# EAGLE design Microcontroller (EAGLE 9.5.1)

## Sheet 1 of 3: Board to Board Headers
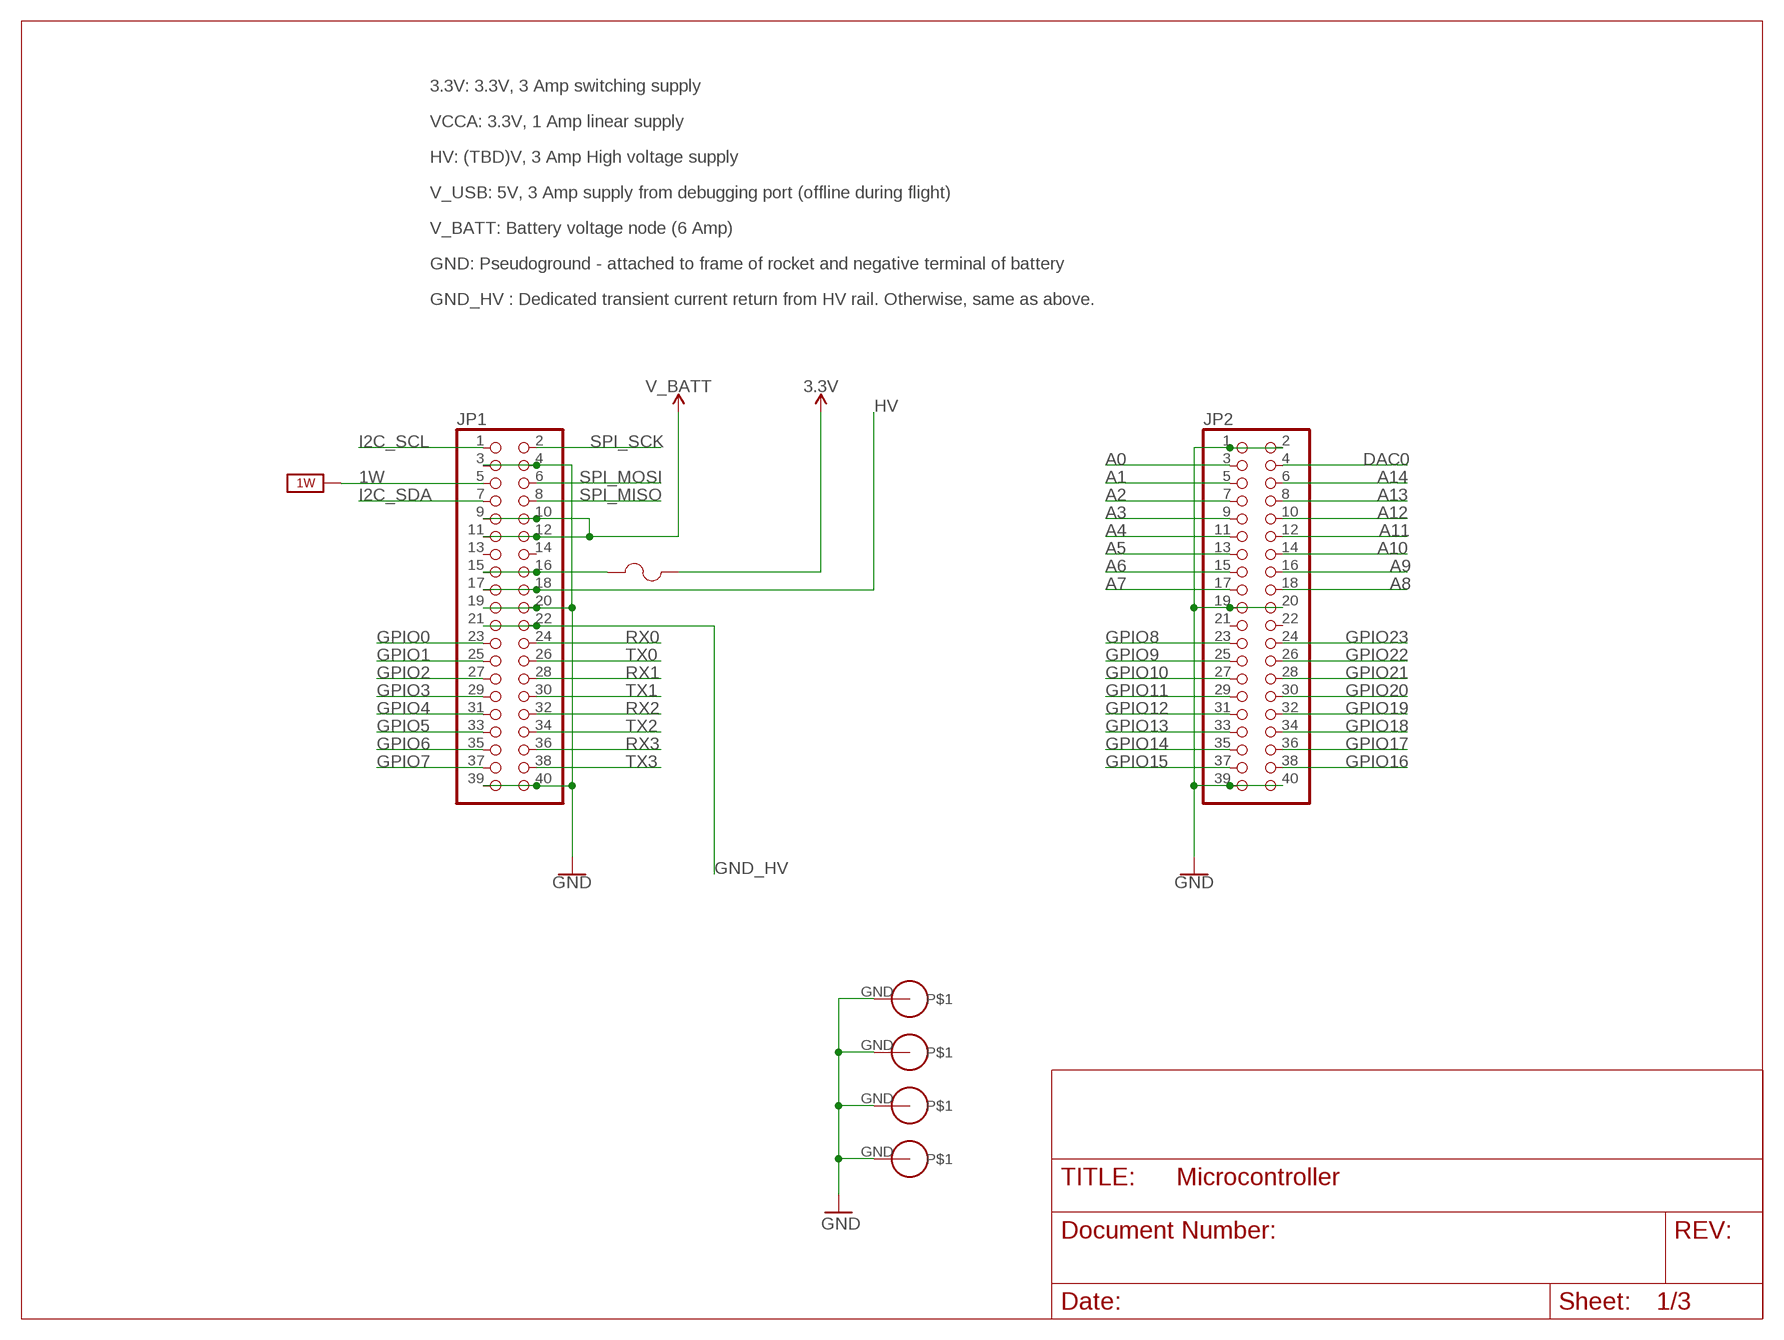
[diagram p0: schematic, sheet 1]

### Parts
F3  0603SFF150F/32-2  [FUS0603_TYCO]
JP1  PINHD-2X20  [2X20]
JP2  PINHD-2X20  [2X20]
U$1  PS/104-MOUNTING-HOLE  [PC/104-MOUNTING-HOLE]
U$2  PS/104-MOUNTING-HOLE  [PC/104-MOUNTING-HOLE]
U$3  PS/104-MOUNTING-HOLE  [PC/104-MOUNTING-HOLE]
U$4  PS/104-MOUNTING-HOLE  [PC/104-MOUNTING-HOLE]

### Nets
1W: JP1.5 ; supply symbol labelled 1W_SUP ; also sheet 3
3.3V: F3.2 ; also sheet 2,3
A0: JP2.3 ; also sheet 2
A1: JP2.5 ; also sheet 2
A2: JP2.7 ; also sheet 2
A3: JP2.9 ; also sheet 2
A4: JP2.11 ; also sheet 2
A5: JP2.13 ; also sheet 2
A6: JP2.15 ; also sheet 2
A7: JP2.17 ; also sheet 2
A8: JP2.18 ; also sheet 2
A9: JP2.16 ; also sheet 2
A10: JP2.14 ; also sheet 2
A11: JP2.12 ; also sheet 2
A12: JP2.10 ; also sheet 2
A13: JP2.8 ; also sheet 2
A14: JP2.6 ; also sheet 2
DAC0: JP2.4 ; also sheet 2
GND: JP1.3 JP1.4 JP1.19 JP1.20 JP1.39 JP1.40 JP2.1 JP2.2 JP2.19 JP2.20 JP2.39 JP2.40 U$1.GND U$2.GND U$3.GND U$4.GND ; also sheet 2,3
GND_HV: JP1.21 JP1.22
GPIO0: JP1.23 ; also sheet 2
GPIO1: JP1.25 ; also sheet 2
GPIO2: JP1.27 ; also sheet 2
GPIO3: JP1.29 ; also sheet 2
GPIO4: JP1.31 ; also sheet 2
GPIO5: JP1.33 ; also sheet 2
GPIO6: JP1.35 ; also sheet 2
GPIO7: JP1.37 ; also sheet 2
GPIO8: JP2.23 ; also sheet 2
GPIO9: JP2.25 ; also sheet 2
GPIO10: JP2.27 ; also sheet 2
GPIO11: JP2.29 ; also sheet 2
GPIO12: JP2.31 ; also sheet 2
GPIO13: JP2.33 ; also sheet 3
GPIO14: JP2.35 ; also sheet 3
GPIO15: JP2.37 ; also sheet 3
GPIO16: JP2.38 ; also sheet 3
GPIO17: JP2.36 ; also sheet 3
GPIO18: JP2.34 ; also sheet 3
GPIO19: JP2.32 ; also sheet 3
GPIO20: JP2.30 ; also sheet 3
GPIO21: JP2.28 ; also sheet 3
GPIO22: JP2.26 ; also sheet 3
GPIO23: JP2.24 ; also sheet 3
HV: JP1.17 JP1.18
I2C_SCL: JP1.1 ; also sheet 2,3
I2C_SDA: JP1.7 ; also sheet 2,3
N$3: F3.1 JP1.15 JP1.16
RX0: JP1.24 ; also sheet 2
RX1: JP1.28 ; also sheet 2
RX2: JP1.32 ; also sheet 2
RX3: JP1.36 ; also sheet 2,3
SPI_MISO: JP1.8 ; also sheet 2,3
SPI_MOSI: JP1.6 ; also sheet 2,3
SPI_SCK: JP1.2 ; also sheet 2,3
TX0: JP1.26 ; also sheet 2
TX1: JP1.30 ; also sheet 2
TX2: JP1.34 ; also sheet 2
TX3: JP1.38 ; also sheet 2,3
V_BATT: JP1.9 JP1.10 JP1.11 JP1.12
Unconnected: JP1.13 JP1.14 JP2.21 JP2.22

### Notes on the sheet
- 3.3V: 3.3V, 3 Amp switching supply
- VCCA: 3.3V, 1 Amp linear supply
- HV: (TBD)V, 3 Amp High voltage supply
- V_USB: 5V, 3 Amp supply from debugging port (offline during flight)
- V_BATT: Battery voltage node (6 Amp)
- GND: Pseudoground - attached to frame of rocket and negative terminal of battery
- GND_HV : Dedicated transient current return from HV rail. Otherwise, same as above.

## Sheet 2 of 3: MCU
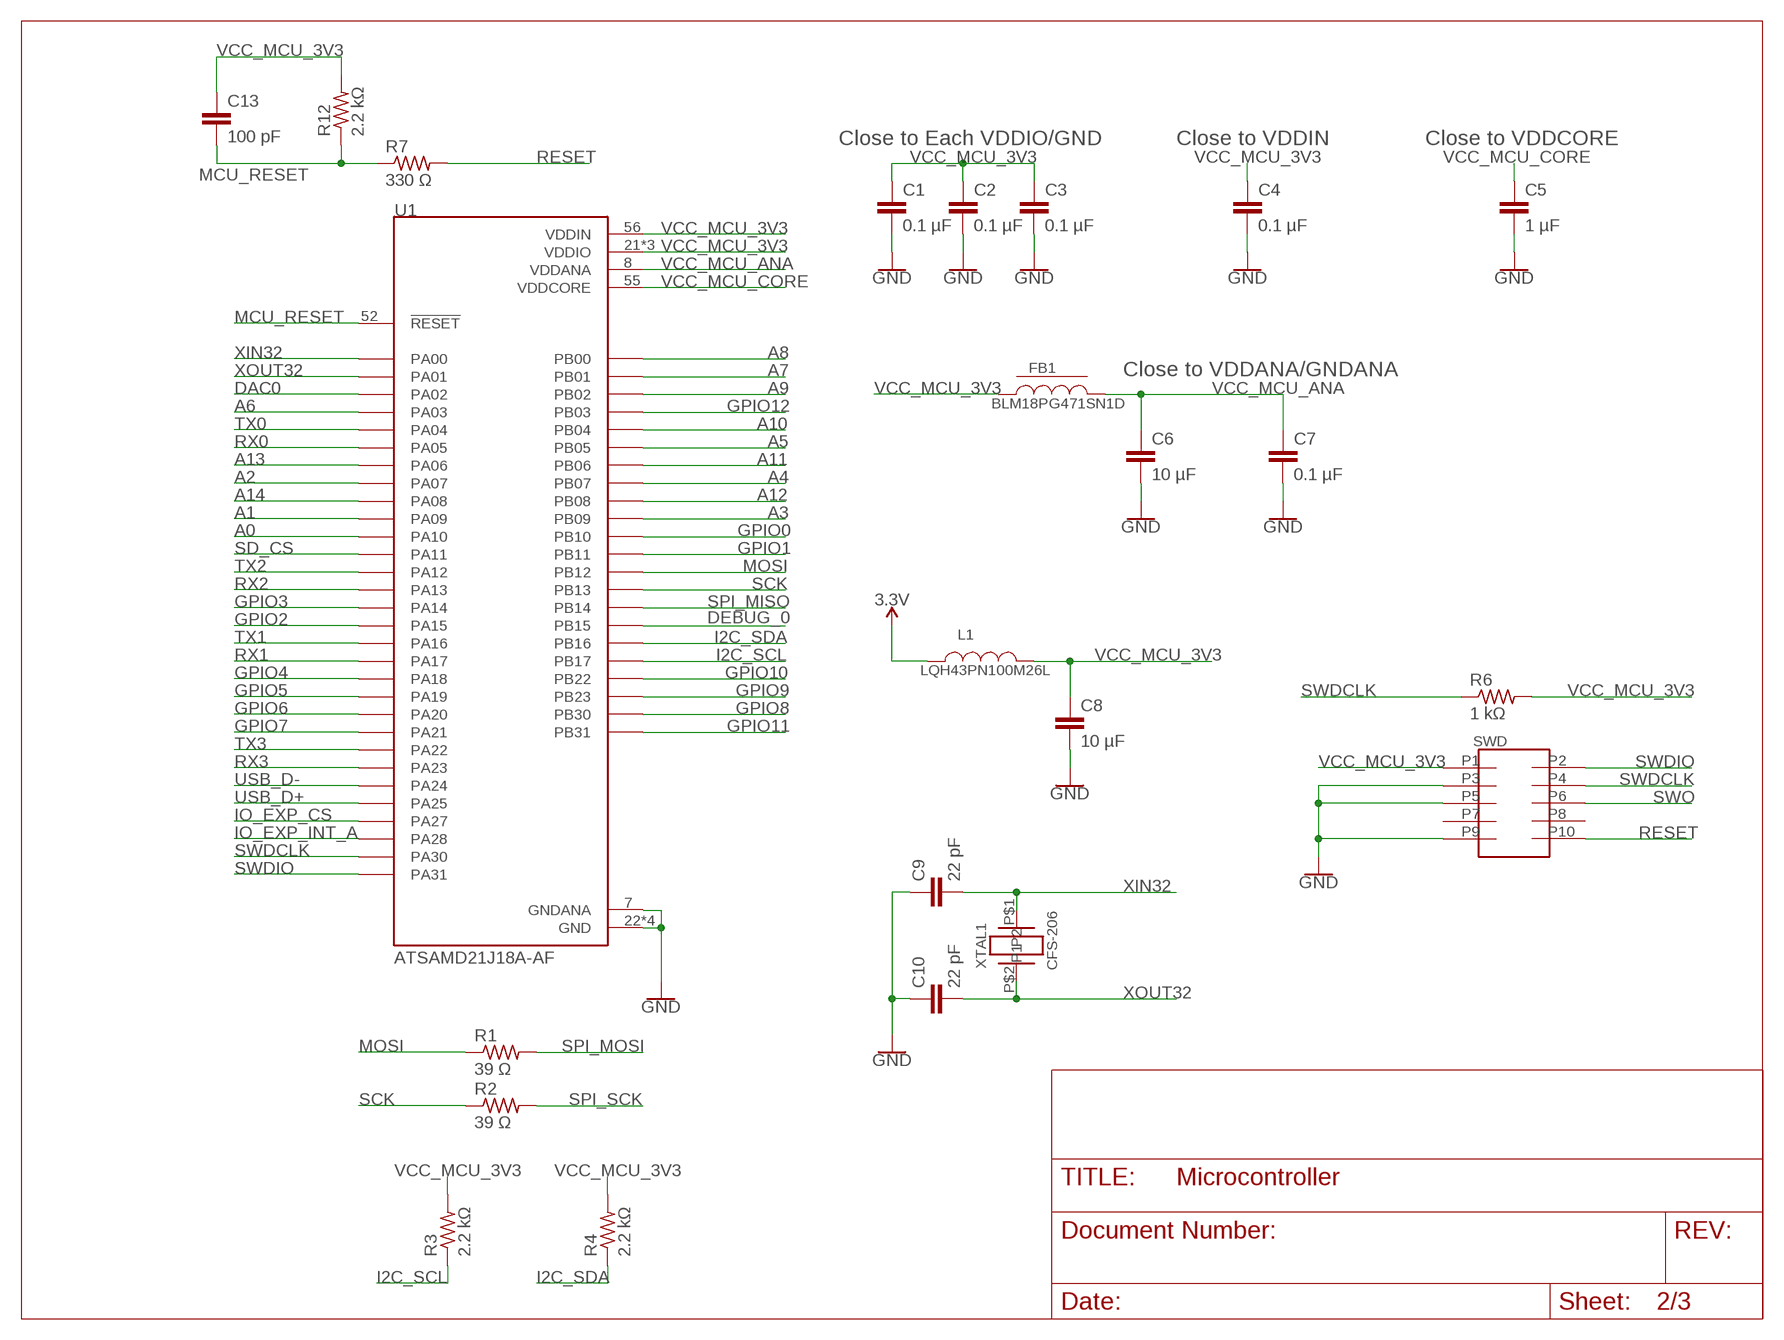
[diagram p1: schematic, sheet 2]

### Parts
C1  0.1 µF  C-EUC0805  [C0805]
C2  0.1 µF  C-EUC0805  [C0805]
C3  0.1 µF  C-EUC0805  [C0805]
C4  0.1 µF  C-EUC0805  [C0805]
C5  1 µF  C-EUC0805  [C0805]
C6  10 µF  C-EUC1206  [C1206]
C7  0.1 µF  C-EUC0805  [C0805]
C8  10 µF  C-EUC1206  [C1206]
C9  22 pF  C-EUC0805  [C0805]
C10  22 pF  C-EUC0805  [C0805]
C13  100 pF  C-EUC0805  [C0805]
FB1  BLM18PG471SN1D  [0603]
L1  LQH43PN100M26L  [LQH43PN100M26L]
R1  39 Ω  R-US_R1206  [R1206]
R2  39 Ω  R-US_R1206  [R1206]
R3  2.2 kΩ  R-US_R1206  [R1206]
R4  2.2 kΩ  R-US_R1206  [R1206]
R6  1 kΩ  R-US_R1206  [R1206]
R7  330 Ω  R-US_R1206  [R1206]
R12  2.2 kΩ  R-US_R1206  [R1206]
SWD  GRPB052VWVN-RC  [GRPB052VWVN-RC]
U1  ATSAMD21J18A-AF  [QFP50P1200X1200X120_64N]
XTAL1  CFS-206  [CFS-206]

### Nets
3.3V: L1.1 ; also sheet 1,3
A0: U1.19(PA10) ; also sheet 1
A1: U1.18(PA09) ; also sheet 1
A2: U1.16(PA07) ; also sheet 1
A3: U1.12(PB09) ; also sheet 1
A4: U1.10(PB07) ; also sheet 1
A5: U1.6(PB05) ; also sheet 1
A6: U1.4(PA03) ; also sheet 1
A7: U1.62(PB01) ; also sheet 1
A8: U1.61(PB00) ; also sheet 1
A9: U1.63(PB02) ; also sheet 1
A10: U1.5(PB04) ; also sheet 1
A11: U1.9(PB06) ; also sheet 1
A12: U1.11(PB08) ; also sheet 1
A13: U1.15(PA06) ; also sheet 1
A14: U1.17(PA08) ; also sheet 1
DAC0: U1.3(PA02) ; also sheet 1
DEBUG_0: U1.28(PB15) ; also sheet 3
GND: C1.2 C2.2 C3.2 C4.2 C5.2 C6.2 C7.2 C8.2 C9.1 C10.1 SWD.P3 SWD.P5 SWD.P9 U1.7(GNDANA) U1.22(GND) U1.33(GND) U1.47(GND) U1.54(GND) ; also sheet 1,3
GPIO0: U1.23(PB10) ; also sheet 1
GPIO1: U1.24(PB11) ; also sheet 1
GPIO2: U1.32(PA15) ; also sheet 1
GPIO3: U1.31(PA14) ; also sheet 1
GPIO4: U1.37(PA18) ; also sheet 1
GPIO5: U1.38(PA19) ; also sheet 1
GPIO6: U1.41(PA20) ; also sheet 1
GPIO7: U1.42(PA21) ; also sheet 1
GPIO8: U1.59(PB30) ; also sheet 1
GPIO9: U1.50(PB23) ; also sheet 1
GPIO10: U1.49(PB22) ; also sheet 1
GPIO11: U1.60(PB31) ; also sheet 1
GPIO12: U1.64(PB03) ; also sheet 1
I2C_SCL: R3.1 U1.40(PB17) ; also sheet 1,3
I2C_SDA: R4.1 U1.39(PB16) ; also sheet 1,3
IO_EXP_CS: U1.51(PA27) ; also sheet 3
IO_EXP_INT_A: U1.53(PA28) ; also sheet 3
MCU_RESET: C13.2 R7.1 R12.1 U1.52(!RESET)
MOSI: R1.1 U1.25(PB12) ; also sheet 3
RESET: R7.2 SWD.P10
RX0: U1.14(PA05) ; also sheet 1
RX1: U1.36(PA17) ; also sheet 1
RX2: U1.30(PA13) ; also sheet 1
RX3: U1.44(PA23) ; also sheet 1,3
SCK: R2.1 U1.26(PB13) ; also sheet 3
SD_CS: U1.20(PA11) ; also sheet 3
SPI_MISO: U1.27(PB14) ; also sheet 1,3
SPI_MOSI: R1.2 ; also sheet 1,3
SPI_SCK: R2.2 ; also sheet 1,3
SWDCLK: R6.1 SWD.P4 U1.57(PA30)
SWDIO: SWD.P2 U1.58(PA31)
SWO: SWD.P6
TX0: U1.13(PA04) ; also sheet 1
TX1: U1.35(PA16) ; also sheet 1
TX2: U1.29(PA12) ; also sheet 1
TX3: U1.43(PA22) ; also sheet 1,3
USB_D+: U1.46(PA25) ; also sheet 3
USB_D-: U1.45(PA24) ; also sheet 3
VCC_MCU_3V3: C1.1 C2.1 C3.1 C4.1 C8.1 C13.1 FB1.1 L1.2 R3.2 R4.2 R6.2 R12.2 SWD.P1 U1.21(VDDIO) U1.34(VDDIO) U1.48(VDDIO) U1.56(VDDIN) ; also sheet 3
VCC_MCU_ANA: C6.1 C7.1 FB1.2 U1.8(VDDANA)
VCC_MCU_CORE: C5.1 U1.55(VDDCORE)
XIN32: C9.2 U1.1(PA00) XTAL1.P$1(P1)
XOUT32: C10.2 U1.2(PA01) XTAL1.P$2(P2)
Unconnected: SWD.P7 SWD.P8

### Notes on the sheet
- Close to Each VDDIO/GND | Close to VDDIN | Close to VDDCORE
- Close to VDDANA/GNDANA

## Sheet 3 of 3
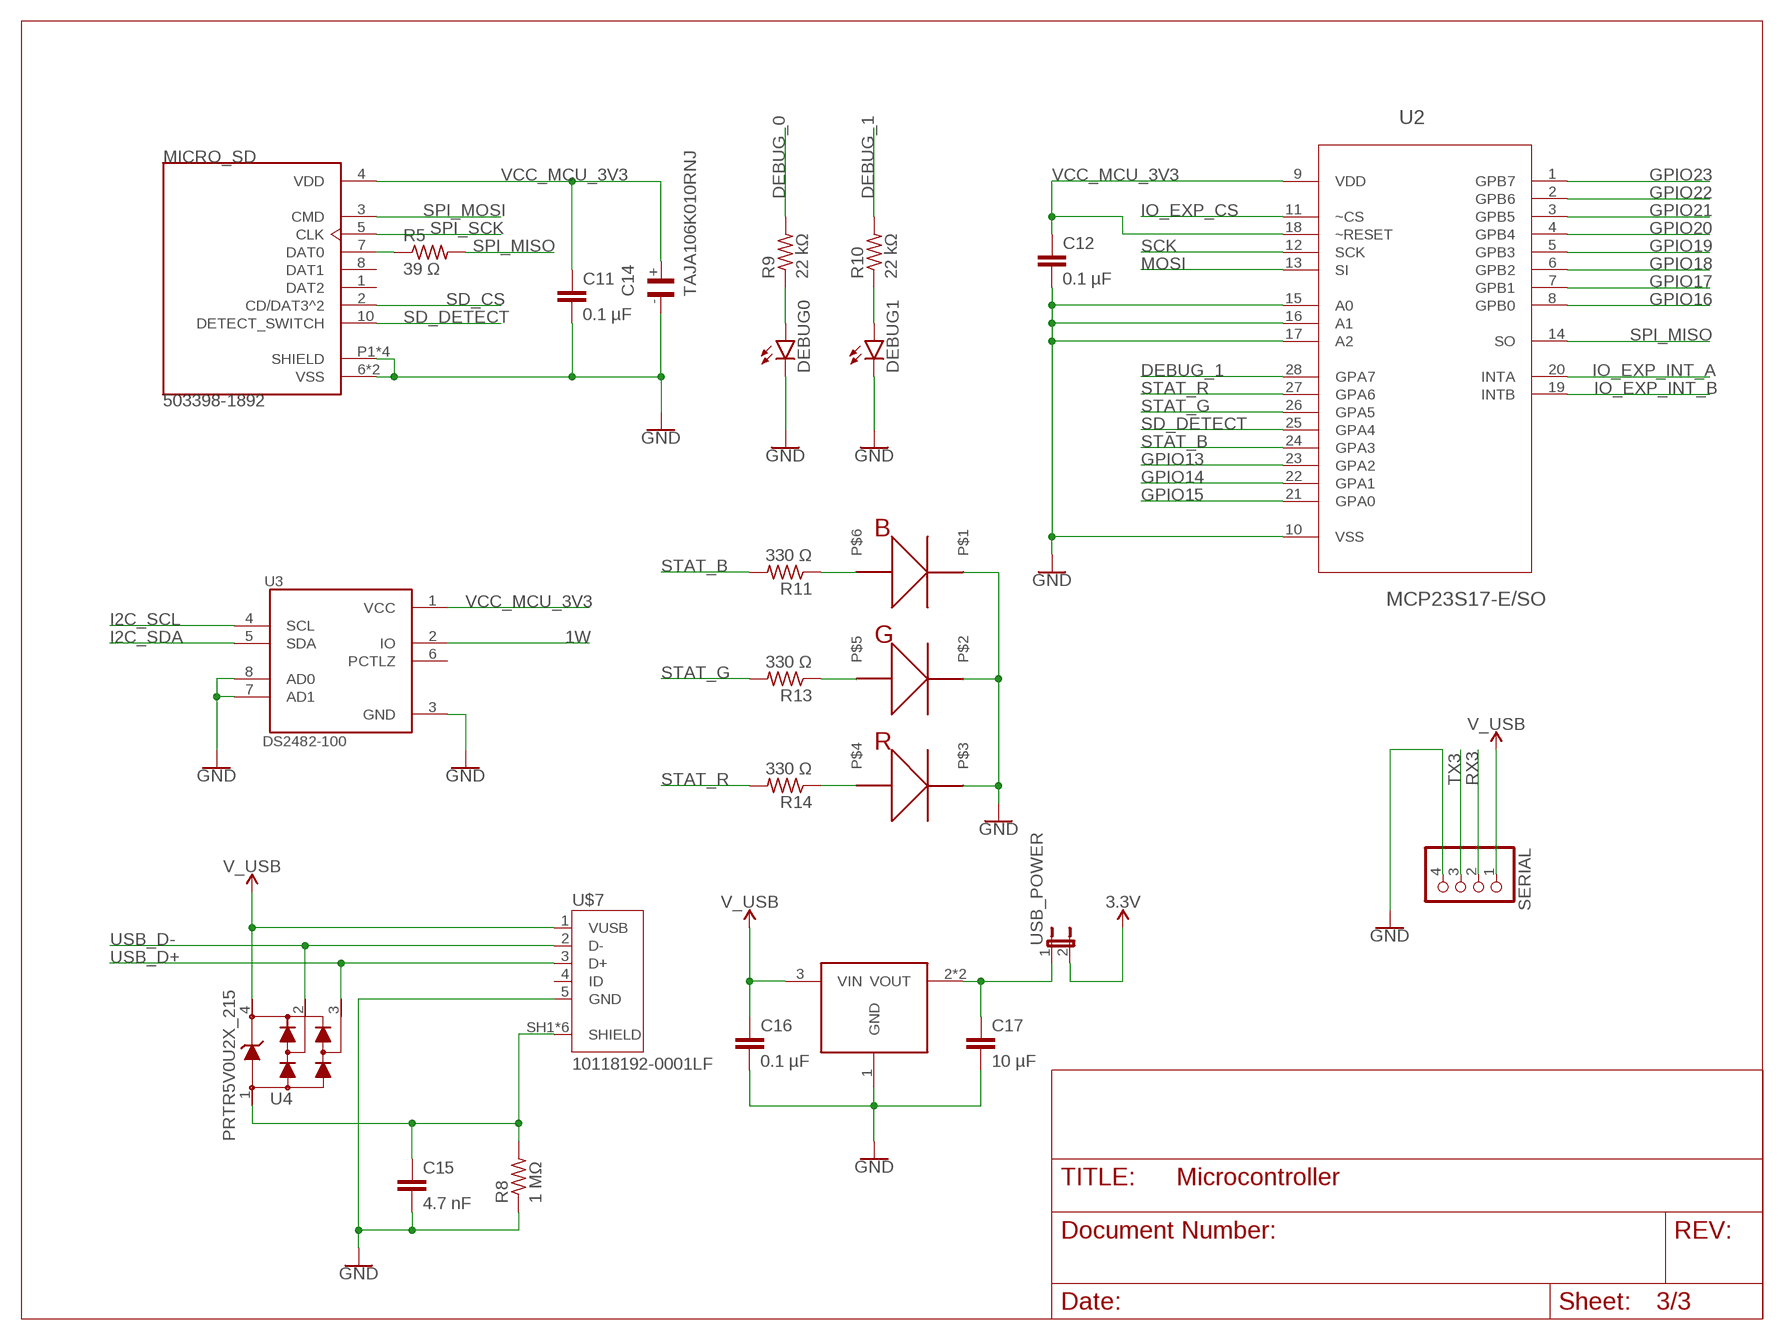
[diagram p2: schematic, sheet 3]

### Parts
C11  0.1 µF  C-EUC0805  [C0805]
C12  0.1 µF  C-EUC0805  [C0805]
C14  TAJA106K010RNJ  [1206-POL]
C15  4.7 nF  C-EUC0805  [C0805]
C16  0.1 µF  C-EUC0805  [C0805]
C17  10 µF  C-EUC1206  [C1206]
DEBUG0  LED3MM  [LED3MM]
DEBUG1  LED3MM  [LED3MM]
MICRO_SD  503398-1892  [MOLEX_503398-1892]
R5  39 Ω  R-US_R1206  [R1206]
R8  1 MΩ  R-US_R1206  [R1206]
R9  22 kΩ  R-US_R1206  [R1206]
R10  22 kΩ  R-US_R1206  [R1206]
R11  330 Ω  R-US_R1206  [R1206]
R13  330 Ω  R-US_R1206  [R1206]
R14  330 Ω  R-US_R1206  [R1206]
SERIAL  PINHD-1X4  [1X04]
STATUS  MSL0402RGB  [MSL0402RGB]
U2  MCP23S17-E/SO  [SOIC28]
U3  DS2482-100  [SOIC8]
U4  PRTR5V0U2X_215  [SOT143B]
U5  LDL1117S33R  [SOT223]
U$7  10118192-0001LF  [10118192-0001LF]
USB_POWER  JP1E  [JP1]

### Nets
1W: U3.2(IO) ; also sheet 1
3.3V: USB_POWER.2 ; also sheet 1,2
DEBUG_0: R9.2 ; also sheet 2
DEBUG_1: R10.2 U2.28(GPA7)
GND: C11.2 C12.2 C14.- C15.2 C16.2 C17.2 DEBUG0.K(C) DEBUG1.K(C) MICRO_SD.6(VSS) MICRO_SD.9(VSS) MICRO_SD.P1(SHIELD) MICRO_SD.P2(SHIELD) MICRO_SD.P3(SHIELD) MICRO_SD.P4(SHIELD) R8.1 SERIAL.4 STATUS.P1 STATUS.P2 STATUS.P3 U2.10(VSS) U2.15(A0) U2.16(A1) U2.17(A2) U3.3(GND) U3.7(AD1) U3.8(AD0) U5.1(GND) U$7.5(GND) ; also sheet 1,2
GPIO13: U2.23(GPA2) ; also sheet 1
GPIO14: U2.22(GPA1) ; also sheet 1
GPIO15: U2.21(GPA0) ; also sheet 1
GPIO16: U2.8(GPB0) ; also sheet 1
GPIO17: U2.7(GPB1) ; also sheet 1
GPIO18: U2.6(GPB2) ; also sheet 1
GPIO19: U2.5(GPB3) ; also sheet 1
GPIO20: U2.4(GPB4) ; also sheet 1
GPIO21: U2.3(GPB5) ; also sheet 1
GPIO22: U2.2(GPB6) ; also sheet 1
GPIO23: U2.1(GPB7) ; also sheet 1
I2C_SCL: U3.4(SCL) ; also sheet 1,2
I2C_SDA: U3.5(SDA) ; also sheet 1,2
IO_EXP_CS: U2.11(~CS) ; also sheet 2
IO_EXP_INT_A: U2.20(INTA) ; also sheet 2
IO_EXP_INT_B: U2.19(INTB)
MOSI: U2.13(SI) ; also sheet 2
N$1: MICRO_SD.7(DAT0) R5.1
N$2: C15.1 R8.2 U4.1 U$7.SH1(SHIELD) U$7.SH2(SHIELD) U$7.SH3(SHIELD) U$7.SH4(SHIELD) U$7.SH5(SHIELD) U$7.SH6(SHIELD)
N$4: DEBUG1.A R10.1
N$5: R11.1 STATUS.P6
N$6: C17.1 U5.2(VOUT) U5.4(VOUT) USB_POWER.1
N$7: DEBUG0.A R9.1
N$8: R13.1 STATUS.P5
N$9: R14.1 STATUS.P4
RX3: SERIAL.2 ; also sheet 1,2
SCK: U2.12(SCK) ; also sheet 2
SD_CS: MICRO_SD.2(CD/DAT3^2) ; also sheet 2
SD_DETECT: MICRO_SD.10(DETECT_SWITCH) U2.25(GPA4)
SPI_MISO: R5.2 U2.14(SO) ; also sheet 1,2
SPI_MOSI: MICRO_SD.3(CMD) ; also sheet 1,2
SPI_SCK: MICRO_SD.5(CLK) ; also sheet 1,2
STAT_B: R11.2 U2.24(GPA3)
STAT_G: R13.2 U2.26(GPA5)
STAT_R: R14.2 U2.27(GPA6)
TX3: SERIAL.3 ; also sheet 1,2
USB_D+: U4.3 U$7.3(D+) ; also sheet 2
USB_D-: U4.2 U$7.2(D-) ; also sheet 2
V_USB: C16.1 SERIAL.1 U4.4 U5.3(VIN) U$7.1(VUSB)
VCC_MCU_3V3: C11.1 C12.1 C14.+ MICRO_SD.4(VDD) U2.9(VDD) U2.18(~RESET) U3.1(VCC) ; also sheet 2
Unconnected: MICRO_SD.1(DAT2) MICRO_SD.8(DAT1) U3.6(PCTLZ) U$7.4(ID)

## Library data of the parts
C1-C13 C15-C17 = rcl:C-EU: CAPACITOR, European symbol; SPICEPREFIX: C
C14 = MCU Board:TAJA106K010RNJ
DEBUG0 DEBUG1 = led:LED: LED
F3 = CU inSpace 2019 Parts:0603SFF150F/32-2; MANUFACTURER_PART_NUMBER: 0603SFF150F322; VENDOR: Littelfuse Inc
FB1 = MCU Board:BLM18PG471SN1D
JP1 JP2 = pinhead:PINHD-2X20: PIN HEADER
L1 = MCU Board:LQH43PN100M26L
MICRO_SD = CUINSPACE_Managed:503398-1892
R1-R14 = rcl:R-US_: RESISTOR, American symbol; SPICEPREFIX: R
SERIAL = pinhead:PINHD-1X4: PIN HEADER
STATUS = MCU Board:MSL0402RGB
SWD = MCU Board:GRPB052VWVN-RC
U1 = MCU Board:ATSAMD21J18A-AF: MCU 32-Bit SAM D21J ARM Cortex M0+ RISC 256KB Flash 3.3V 64-Pin TQFP Tray; AVAILABILITY: Unavailable; DESCRIPTION: MCU 32-Bit SAM D21J ARM Cortex M0+ RISC 256KB Flash 3.3V 64-Pin TQFP Tray; MF: Microchip; MP: ATSAMD21J18A-AF; PACKAGE: TQFP-64 Microchip; PRICE: None
U2 = MCU Board:MCP23S17-E/SO
U3 = MCU Board:DS2482-100
U4 = MCU Board:PRTR5V0U2X_215
U5 = MCU Board:LDL1117S33R
U$1-U$4 = CU inSpace 2019 Parts:PS/104-MOUNTING-HOLE: Mounting hole for PC/104 board.
U$7 = MCU Board:10118192-0001LF
USB_POWER = jumper:JP1E: JUMPER
XTAL1 = MCU Board:CFS-206

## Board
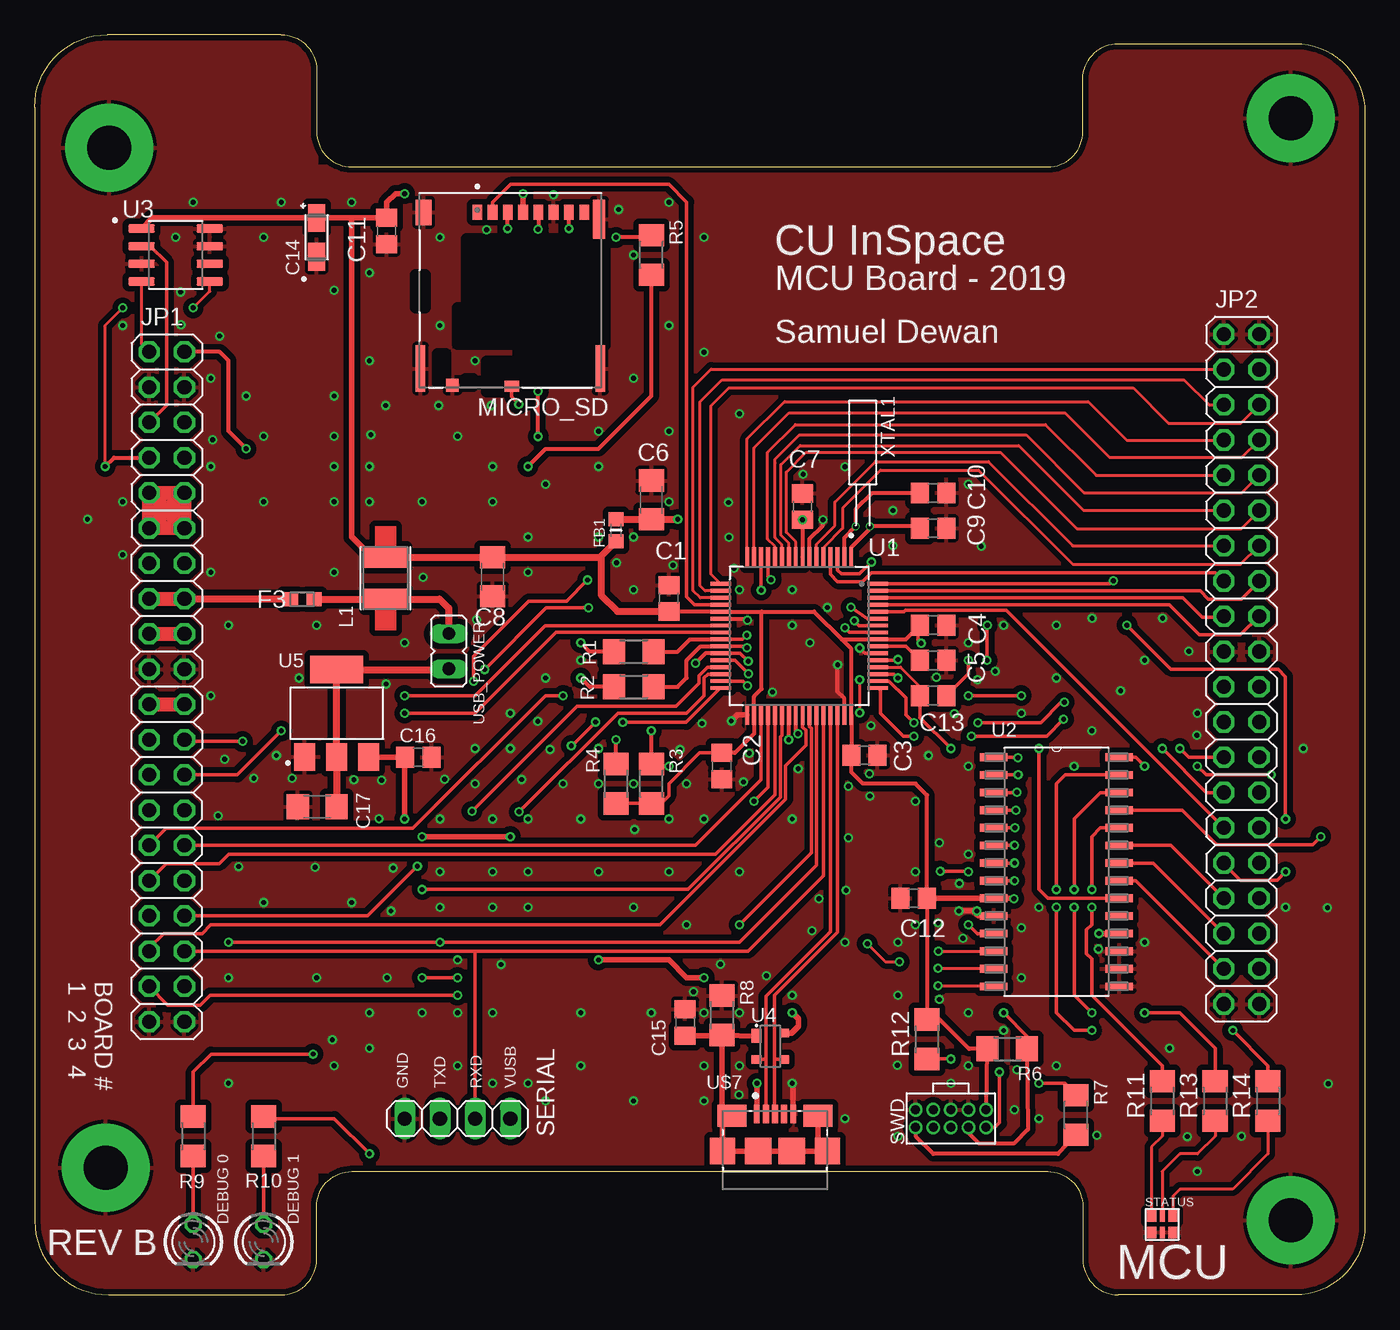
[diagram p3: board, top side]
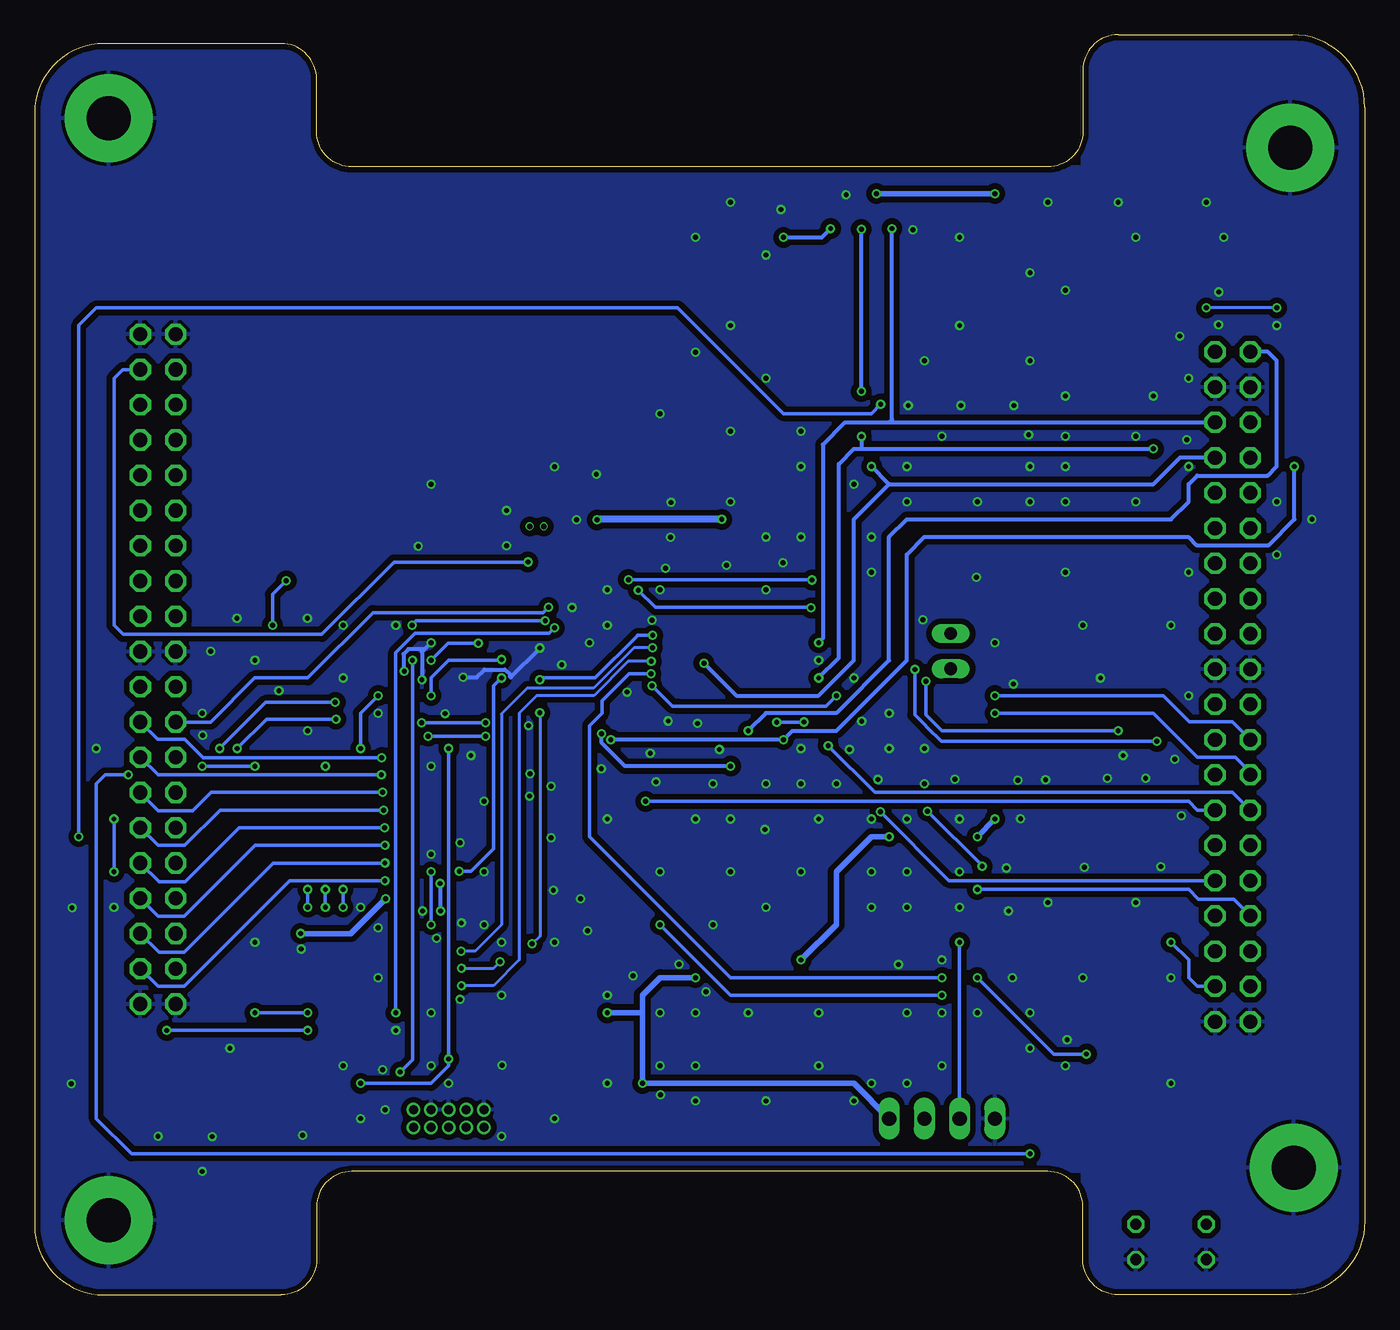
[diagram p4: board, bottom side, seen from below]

Size 95.89 x 90.81 mm. Coordinates in mm from the lower left corner, seen from the top.
Outline: 0,85.57 0,5.33 arc90 5.33,0 17.78,0 arc90 20.32,2.54 20.32,6.35 arc-90 22.86,8.89 73.03,8.89 arc-90 75.56,6.35 75.56,2.54 arc90 78.11,0 90.89,0 arc90 95.89,5 95.89,85.17 arc90 90.89,90.17 78.11,90.17 arc90 75.56,87.63 75.56,83.82 arc-90 73.03,81.28 22.86,81.28 arc-90 20.32,83.82 20.32,88.27 arc90 17.78,90.81 5.23,90.81 arc90 0,85.57
Copper layers (1*16): Top 0.035mm / dielectric 1.5mm / Bottom 0.035mm
Design rules "JLCPCB *": minimum track width 3.5mil, minimum drill 0.2mm, track to track 5mil, track to pad 5mil, pad to pad 5mil, via to via 5mil, smd to smd 0mil, copper to edge 10mil, drill to drill 10mil, minimum pad ring 3mil, minimum via ring 6mil, stop-mask expansion 2mil, vias tented up to drill 25mil, thermal gap 10mil

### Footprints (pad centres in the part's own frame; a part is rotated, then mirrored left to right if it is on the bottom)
C0805 = smd 1.3 x 1.5: 1 -0.95,0; 2 0.95,0
C1206 = smd 1.6 x 1.8: 1 -1.4,0; 2 1.4,0
1206-POL = smd 2 x 1.2: + 1.4,0; - -1.4,0
LED3MM = drill 0.813 octagon: A -1.27,0; K 1.27,0
FUS0603_TYCO = smd 1.092 x 0.991: 1 -0.851,0; 2 0.851,0
0603 = smd 1 x 1.1: 1 -0.794,0; 2 0.794,0
2X20 = drill 1.016 octagon: 1 -24.13,-1.27; 2 -24.13,1.27; 3 -21.59,-1.27; 4 -21.59,1.27; 5 -19.05,-1.27; 6 -19.05,1.27; 7 -16.51,-1.27; 8 -16.51,1.27; 9 -13.97,-1.27; 10 -13.97,1.27; 11 -11.43,-1.27; 12 -11.43,1.27; 13 -8.89,-1.27; 14 -8.89,1.27; 15 -6.35,-1.27; 16 -6.35,1.27; 17 -3.81,-1.27; 18 -3.81,1.27; 19 -1.27,-1.27; 20 -1.27,1.27; 21 1.27,-1.27; 22 1.27,1.27; 23 3.81,-1.27; 24 3.81,1.27; 25 6.35,-1.27; 26 6.35,1.27; 27 8.89,-1.27; 28 8.89,1.27; 29 11.43,-1.27; 30 11.43,1.27; 31 13.97,-1.27; 32 13.97,1.27; 33 16.51,-1.27; 34 16.51,1.27; 35 19.05,-1.27; 36 19.05,1.27; 37 21.59,-1.27; 38 21.59,1.27; 39 24.13,-1.27; 40 24.13,1.27
LQH43PN100M26L = smd 1.5 x 3: 1 -1.5,0; 2 1.5,0
MOLEX_503398-1892 = smd 0.7 x 1.1: 1 -3.65,6.895; 2 -2.55,6.895; 3 -1.45,6.895; 4 -0.35,6.895; 5 0.75,6.895; 6 1.85,6.895; 7 2.95,6.895; 8 4.05,6.895 | smd 0.9 x 0.93: 9 -5.44,-5.57 | smd 1.05 x 0.78: 10 -1.175,-5.645 | smd 1.14 x 1.83: P1 -7.53,6.88 | smd 0.86 x 2.8: P2 5.13,6.395 | smd 0.7 x 3.33: P3 -7.75,-4.37; P4 5.21,-4.37
R1206 = smd 1.6 x 1.803: 1 -1.422,0; 2 1.422,0
1X04 = drill 1.016 long: 1 -3.81,0; 2 -1.27,0; 3 1.27,0; 4 3.81,0
MSL0402RGB = smd 0.67 x 0.83: P1 0.77,-0.585; P3 -0.77,-0.585; P4 0.77,0.585; P6 -0.77,0.585 | smd 0.37 x 0.83: P2 0,-0.585; P5 0,0.585
GRPB052VWVN-RC = drill 0.65 pad 0.9: P1 2.54,0.635; P2 2.54,-0.635; P3 1.27,0.635; P4 1.27,-0.635; P5 0,0.635; P6 0,-0.635; P7 -1.27,0.635; P8 -1.27,-0.635; P9 -2.54,0.635; P10 -2.54,-0.635
QFP50P1200X1200X120_64N = smd 1.47 x 0.28: 1 -5.67,3.75; 2 -5.67,3.25; 3 -5.67,2.75; 4 -5.67,2.25; 5 -5.67,1.75; 6 -5.67,1.25; 7 -5.67,0.75; 8 -5.67,0.25; 9 -5.67,-0.25; 10 -5.67,-0.75; 11 -5.67,-1.25; 12 -5.67,-1.75; 13 -5.67,-2.25; 14 -5.67,-2.75; 15 -5.67,-3.25; 16 -5.67,-3.75; 33 5.67,-3.75; 34 5.67,-3.25; 35 5.67,-2.75; 36 5.67,-2.25; 37 5.67,-1.75; 38 5.67,-1.25; 39 5.67,-0.75; 40 5.67,-0.25; 41 5.67,0.25; 42 5.67,0.75; 43 5.67,1.25; 44 5.67,1.75; 45 5.67,2.25; 46 5.67,2.75; 47 5.67,3.25; 48 5.67,3.75 | smd 0.28 x 1.47: 17 -3.75,-5.67; 18 -3.25,-5.67; 19 -2.75,-5.67; 20 -2.25,-5.67; 21 -1.75,-5.67; 22 -1.25,-5.67; 23 -0.75,-5.67; 24 -0.25,-5.67; 25 0.25,-5.67; 26 0.75,-5.67; 27 1.25,-5.67; 28 1.75,-5.67; 29 2.25,-5.67; 30 2.75,-5.67; 31 3.25,-5.67; 32 3.75,-5.67; 49 3.75,5.67; 50 3.25,5.67; 51 2.75,5.67; 52 2.25,5.67; 53 1.75,5.67; 54 1.25,5.67; 55 0.75,5.67; 56 0.25,5.67; 57 -0.25,5.67; 58 -0.75,5.67; 59 -1.25,5.67; 60 -1.75,5.67; 61 -2.25,5.67; 62 -2.75,5.67; 63 -3.25,5.67; 64 -3.75,5.67
SOIC28 = smd 1.981 x 0.559: 1 -4.521,8.255; 2 -4.521,6.985; 3 -4.521,5.715; 4 -4.521,4.445; 5 -4.521,3.175; 6 -4.521,1.905; 7 -4.521,0.635; 8 -4.521,-0.635; 9 -4.521,-1.905; 10 -4.521,-3.175; 11 -4.521,-4.445; 12 -4.521,-5.715; 13 -4.521,-6.985; 14 -4.521,-8.255; 15 4.521,-8.255; 16 4.521,-6.985; 17 4.521,-5.715; 18 4.521,-4.445; 19 4.521,-3.175; 20 4.521,-1.905; 21 4.521,-0.635; 22 4.521,0.635; 23 4.521,1.905; 24 4.521,3.175; 25 4.521,4.445; 26 4.521,5.715; 27 4.521,6.985; 28 4.521,8.255
SOIC8 = smd 1.91 x 0.6: 1 -2.46,1.905; 2 -2.46,0.635; 3 -2.46,-0.635; 4 -2.46,-1.905; 5 2.46,-1.905; 6 2.46,-0.635; 7 2.46,0.635; 8 2.46,1.905
SOT143B = smd 1 x 0.7: 1 -0.75,-1 | smd 0.6 x 0.7: 2 0.95,-1; 3 0.95,1; 4 -0.95,1
SOT223 = smd 1.5 x 2: 1 -2.3,-3.15; 2 0,-3.15; 3 2.3,-3.15 | smd 3.8 x 2: 4 0,3.15
PC/104-MOUNTING-HOLE = drill 3.175 pad 6.35: GND 0,0
10118192-0001LF = smd 0.4 x 1.35: 1 -1.3,2.54; 2 -0.65,2.54; 3 0,2.54; 4 0.65,2.54; 5 1.3,2.54 | smd 2.1 x 1.6: SH1 -3.1,2.415; SH2 3.1,2.415 | smd 1.8 x 1.9: SH3 -3.8,-0.135; SH6 3.8,-0.135 | smd 1.9 x 1.9: SH4 -1.2,-0.135; SH5 1.2,-0.135
JP1 = drill 0.914 long: 1 0,-1.27; 2 0,1.27
CFS-206 = drill 0.381: P$1 3.048,0.508; P$2 3.048,-0.508

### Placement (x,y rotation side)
C1  45.72,50.19 90 top
C2  49.53,38.1 270 top
C3  59.82,38.89 0 top
C4  64.77,48.26 0 top
C5  64.77,45.72 0 top
C6  44.45,57.28 90 top
C7  55.35,56.79 90 top
C8  33.02,51.74 270 top
C9  64.77,55.24 180 top
C10  64.77,57.78 180 top
C11  25.37,76.66 270 top
C12  63.37,28.57 180 top
C13  64.77,43.18 180 top
C14  20.32,76.2 90 top
C15  46.89,19.63 90 top
C16  27.66,38.73 0 top
C17  20.37,35.18 180 top
DEBUG0  11.43,3.81 270 top
DEBUG1  16.51,3.81 270 top
F3  19.29,50.13 0 top
FB1  41.91,55.09 90 top
JP1  9.53,43.81 270 top
JP2  87,45.09 270 top
L1  25.3,51.64 90 top
MICRO_SD  35.56,71.12 0 top
R1  43.18,46.35 180 top
R2  43.18,43.81 180 top
R3  44.45,36.83 270 top
R4  41.91,36.83 270 top
R5  44.45,74.93 270 top
R6  70.1,17.73 180 top
R7  75.06,12.95 270 top
R8  49.56,20.14 270 top
R9  11.43,11.43 90 top
R10  16.51,11.43 90 top
R11  81.28,13.97 90 top
R12  64.31,18.41 90 top
R13  85.09,13.97 90 top
R14  88.9,13.97 90 top
SERIAL  30.48,12.7 180 top
STATUS  81.28,5.08 0 top
SWD  66.04,12.7 0 top
U1  55.11,47.48 270 top
U2  73.66,30.48 0 top
U3  10.16,74.93 0 top
U4  53.04,17.91 270 top
U5  21.77,41.91 0 top
U$1  5.36,82.65 0 top
U$2  90.55,84.79 0 top
U$3  5.13,9.17 0 top
U$4  90.55,5.36 0 top
U$7  53.37,10.49 0 top
USB_POWER  29.84,46.38 0 top
XTAL1  59.69,58.42 270 top

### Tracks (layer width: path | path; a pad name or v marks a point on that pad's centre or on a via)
1W
  Top 0.254: JP1.5 9.5,64.11 9.5,74.4 8.33,75.56 U3.2
3.3V
  Top 0.508: F3.2 25.29,50.13 L1.1 29.19,50.14 29.84,49.48 USB_POWER.2
A0
  Top 0.203: U1.19 47.99,50.23 47.47,50.75 47.47,65.41 48.77,66.7 85.7,66.7 JP2.3
A1
  Top 0.203: U1.18 48.33,50.73 47.95,51.1 47.95,64.34 49.55,65.94 82.86,65.94 84.66,64.14 JP2.5
A2
  Top 0.203: U1.16 51.36,61.67 54.05,64.36 75.95,64.36 78.74,61.57 85.7,61.57 JP2.7
A3
  Top 0.203: U1.12 53.36,53.93 52.83,54.46 52.83,60.71 54.84,62.71 72.87,62.71 76.53,59.05 JP2.9
A4
  Top 0.203: U1.10 54.36,54.17 53.8,54.74 53.8,59.82 55.17,61.19 70.94,61.19 75.59,56.54 85.7,56.54 JP2.11
A5
  Top 0.203: U1.6 56.36,54.1 57.68,55.42 57.68,57.12 60.6,60.05 68.76,60.05 74.83,53.98 JP2.13
A6
  Top 0.254: U1.4 57.36,51.91 57.89,51.38 59.66,51.38 60.33,52.05 85.11,52.05 JP2.15
A7
  Top 0.254: U1.62 82.77,50.23 84.18,48.82 85.65,48.82 JP2.17
A8
  Top 0.254: U1.61 81.79,49.73 83.97,47.55 86.92,47.55 JP2.18
A9
  Top 0.254: U1.63 84.02,50.73 84.61,50.14 86.97,50.14 JP2.16
A10
  Top 0.203: U1.5 56.86,53.85 58.24,55.23 58.24,56.69 60.98,59.44 68.05,59.44 74.85,52.63 86.92,52.63 JP2.14
A11
  Top 0.203: U1.9 54.86,54.26 54.18,54.94 54.18,59.28 55.6,60.71 69.62,60.71 75.13,55.19 86.97,55.19 88.27,56.49 JP2.12
A12
  Top 0.203: U1.11 53.86,54.06 53.37,54.56 53.37,59.94 53.37,60.22 55.12,61.98 71.48,61.98 75.64,57.81 87.02,57.81 JP2.10
A13
  Top 0.203: U1.15 51.86,61.03 54.38,63.55 74.27,63.55 77.47,60.35 87.02,60.35 JP2.8
A14
  Top 0.203: U1.17 48.74,51.93 48.74,64.06 50.04,65.35 79.2,65.35 81.74,62.81 86.94,62.81 JP2.6
DAC0  (via drill 0.35)
  Top 0.254: U1.3 57.86,52.22 58.14,51.94 59.46,51.94 v60.33,52.81
  Bottom 0.254: JP2.4 89.53,66.67 90.17,66.04 90.17,48.26 89.51,47.6 75.18,47.6 69.98,52.81 v60.33,52.81
DEBUG_0  (via drill 0.35)
  Top 0.254: v30.48,22.86 v27.94,22.86 | U1.28 50.49,45.73 v51.46,44.76 | R9.2 11.43,16.06 12.72,17.35 v20.07,17.35
  Bottom 0.254: v30.48,22.86 45.72,22.86 55.88,33.02 55.88,41.02 54.99,41.91 54.99,42.8 53.03,44.76 v51.46,44.76 | v27.94,22.86 22.43,17.35 v20.07,17.35
DEBUG_1  (via drill 0.35)
  Top 0.254: R10.2 16.66,12.7 21.59,12.7 v24.13,10.16 | v89.13,37.47 84.45,37.47 v83.82,38.1 | U2.28 79.38,38.73 v80.01,38.1
  Bottom 0.254: v24.13,10.16 88.9,10.16 91.44,12.7 91.44,36.83 90.81,37.47 v89.13,37.47 | v83.82,38.1 v80.01,38.1
GND  (via drill 0.35)
  Top 0.254: U1.54 59.85,46.23 v59.47,46.61
  Top 0.305: U1.47 58.36,42.98 57.89,43.46 v57.89,45.39 | U1.22 51.27,48.73 v51.38,48.62 | U1.7 55.86,54.47 56.82,55.42 v56.82,55.85
  Top 0.406: U2.10 68.02,27.3 67.64,27.69 66.65,27.69 v66.62,27.66 | U$7.5 54.66,15.19 v54.61,15.24 | v50.22,41.35 50.67,41.81 U1.33
  Bottom 0.305: v59.47,46.61 61.58,44.5 61.62,44.55 61.62,44.7 61.98,45.06 63.47,45.06 64.02,44.5 v65.01,44.5 | v67.97,44.32 67.97,46.33 v67.31,46.99 67.77,46.53 68.94,46.53 69.29,46.18 69.29,44.98 v69.24,44.93 | v66.62,27.66 66.62,29.62 v66.65,29.64
  other vias: 16.51,76.2 24.13,73.66 46.02,52.58 43.18,54.61 43.18,50.8 41.94,52.76 40.64,54.61 40.64,59.69 45.72,57.15 50.8,50.8 54.61,50.8 57.15,49.53 54.61,48.26 55.88,46.99 60.27,41.02 60.17,37.54 60.2,35.94 58.67,36.65 58.67,32.94 58.5,29.16 58.42,25.4 62.23,25.4 63.5,35.56 63.5,30.48 73.66,48.26 80.01,45.72 83.82,41.91 81.31,48.74 76.23,48.74 93.19,27.89 93.24,15.21 64.44,38.86 65.23,32.59 65.13,26.8 66.9,25.7 71.12,26.44 72.39,27.94 63.5,26.67 62.23,21.59 67.31,20.32 71.12,22.86 80.01,25.4 72.39,12.7 70.61,13.34 70.82,16.21 67.31,16.51 66.04,15.24 62.2,16.54 56.54,28.55 53.19,43.43 48.11,41.17 46.53,39.29 51.51,39.01 46.99,36.83 51.1,36.96 48.26,34.29 45.72,34.29 39.37,34.29 43.23,33.53 35.56,34.29 38.1,36.83 40.64,39.37 40.64,36.83 43.18,36.83 35.56,30.48 40.64,30.48 45.72,30.48 33.02,30.48 29.21,34.29 34.29,41.91 29.21,30.48 31.75,36.83 34.29,39.37 36.27,41.33 37.16,39.29 35.1,37.13 33.02,34.29 31.75,39.37 29.54,37.16 23.01,37.11 25.02,37.08 24.82,34.32 13.23,34.52 15.8,37.24 18.57,37.24 17.42,38.86 66.3,41.88 67.31,58.42 61.87,56.52 61.87,53.98 69.85,48.26 71.12,41.91 73.66,44.45 67.92,27.66 76.2,40.64 35.56,52.07 36.83,44.45 35.56,54.61 33.02,57.15 27.94,57.15 24.13,57.15 21.59,57.15 16.51,57.15 12.7,59.69 6.35,57.15 6.35,53.34 3.81,55.88 12.7,52.07 13.97,48.26 20.32,48.26 21.59,52.07 31.85,48.64 27.99,51.71 26.67,46.99 25.32,44.02 19.05,44.45 12.7,43.18 13.69,38.58 14.71,30.86 20.22,30.81 25.83,30.76 22.86,28.27 16.51,28.27 25.68,27.66 29.21,27.94 33.02,27.94 35.56,27.94 43.18,27.94 46.99,26.67 50.8,30.48 54.61,34.29 44.45,20.32 50.8,16.51 50.77,14.43 48.26,13.97 48.26,16.51 43.18,13.97 36.83,13.97 35.56,15.24 39.37,16.51 39.37,20.32 33.02,20.32 33.63,23.8 30.48,20.32 30.48,16.51 33.02,15.24 27.94,20.32 24.13,20.32 24.13,17.78 21.46,18.39 21.59,16.51 13.97,15.24 13.97,22.86 25.4,22.86 20.32,22.86 30.48,24.13 33.02,59.69 21.59,59.69 24.13,59.69 24.23,61.98 21.59,61.87 16.51,61.87 30.48,61.87 12.83,61.62 36.83,58.42 40.64,62.23 32.92,64.08 29.11,64.08 25.3,64.08 21.59,64.77 21.59,72.39 24.13,67.31 22.86,78.74 17.78,78.74 11.43,78.74 10.16,76.2 10.54,69.9 6.35,69.85 29.21,69.85 29.21,76.2 32.56,76.76 37.39,79.27 42.09,78.21 45.72,78.74 43.18,74.93 43.18,66.04 45.72,69.85 48.26,76.2 45.72,62.23 50.42,52.35 54.61,21.59 52.76,22.99 56.03,26.24 49.43,23.83 47.5,21.84 48.26,20.32 50.8,20.32 73.66,16.51 76.58,11.51 15.24,64.77 12.7,66.04 13.34,69.09 31.75,67.31 55.04,37.9 69.85,19.05 62.23,11.43 58.42,12.7 10.52,72.26 68.23,53.95 78.28,43.54 58.42,59.66 55.4,59.13 50.04,54.58 50.01,57.1 50.8,63.5 48.26,67.92 83.77,40.31 39.37,45.72 65.23,21.29 67.31,38.1 67.31,31.75 74.93,38.1 81.81,17.75 83.08,11.4 87,11.43 91.44,39.37 83.21,46.38 90.17,27.94 83.82,8.89 76.68,24.92
  pour Top (isolate 0.406): 0,91.44 0,0 20.32,0 20.32,8.89 74.93,8.89 74.93,0 96.52,0 96.52,90.17 74.93,90.17 74.93,81.28 20.32,81.28 20.32,91.44
  pour Bottom (isolate 0.406): 0,91.44 0,0 20.32,0 20.32,8.89 74.93,8.89 74.93,0 96.52,0 96.52,90.17 74.93,90.17 74.93,81.28 20.32,81.28 20.32,91.44
GND_HV
  Top 1.016: JP1.21 JP1.22
GPIO0  (via drill 0.35)
  Top 0.254: U1.23 36.8,48.23 31.75,43.18 v26.67,43.18
  Bottom 0.254: v26.67,43.18 14.53,43.18 12.65,41.3 9.55,41.3 JP1.23
GPIO1  (via drill 0.35)
  Top 0.254: U1.24 37.57,47.73 31.75,41.91 v26.67,41.91
  Bottom 0.254: v26.67,41.91 15.24,41.91 12.06,38.73 9.35,38.73 8.26,37.64 JP1.25
GPIO2  (via drill 0.35)
  Top 0.254: U1.32 46.96,41.25 v42.39,41.25 | v40.44,41.27 38.73,39.57 v38.68,39.57
  Bottom 0.254: v42.39,41.25 40.46,41.25 v40.44,41.27 | v38.68,39.57 35.33,36.22 9.55,36.22 JP1.27
GPIO3  (via drill 0.35)
  Top 0.254: v38.1,43.18 36.83,43.18 27.25,33.6 9.47,33.6 JP1.29 | U1.31 51.05,44.23 v51.38,43.89
  Bottom 0.254: v38.1,43.18 38.86,42.42 49.53,42.42 49.73,42.42 49.91,42.42 v51.38,43.89
GPIO4
  Top 0.254: JP1.31 9.47,31.06 13.28,31.06 13.97,31.75 49.08,31.75 53.36,36.03 U1.37
GPIO5  (via drill 0.35)
  Top 0.254: U1.38 53.86,40.33 53.74,40.21 53.74,35.87 47.08,29.21 v27.94,29.21
  Bottom 0.254: v27.94,29.21 12.7,29.21 11.99,28.5 9.45,28.5 JP1.33
GPIO6
  Top 0.254: U1.41 55.36,40.91 55.6,40.68 55.6,39.6 54.12,38.12 54.12,35.72 45.08,26.67 12.7,26.67 12.06,26.04 9.3,26.04 8.26,24.99 JP1.35
GPIO7  (via drill 0.35)
  Top 0.254: U1.42 55.86,40.95 55.98,40.84 55.98,31.85 v50.8,26.67 | v30.48,21.59 12.65,21.59 11.94,20.88 9.6,20.88 JP1.37
  Bottom 0.254: v50.8,26.67 45.72,21.59 v30.48,21.59
GPIO8  (via drill 0.35)
  Top 0.254: U1.59 60.02,48.73 v58.84,49.53
  Bottom 0.254: JP2.23 83.19,41.27 80.01,44.45 76.2,44.45 71.49,49.16 59.22,49.16 v58.84,49.53
GPIO9  (via drill 0.35)
  Top 0.254: v74.22,42.7 73.99,42.7 72.52,41.22 v68,41.22 | JP2.25 83.19,38.73 v82.55,39.37 | U1.50 61.59,44.23 62.79,43.03 62.79,41.8 v63.37,41.22
  Bottom 0.254: v74.22,42.7 79.22,42.7 v82.55,39.37 | v63.37,41.22 v67.99,41.22 v68,41.22
GPIO10  (via drill 0.35)
  Top 0.254: U1.49 60.96,43.55 60.96,41.91 62.61,40.26 v63.37,40.26 | v81.28,39.37 84.45,36.2 JP2.27 | v67.51,40.26 72.95,40.26 v74.17,41.48
  Bottom 0.254: v74.17,41.48 79.17,41.48 v81.28,39.37 | v63.37,40.26 v67.51,40.26
GPIO11
  Top 0.254: U1.60 62.66,49.23 62.78,49.35 70.03,49.35 JP2.29
GPIO12  (via drill 0.35)
  Top 0.254: U1.64 77.52,51.23 v77.75,51.46 | v78.74,48.26 81.92,45.09 89.64,45.09 90.17,44.55 v90.17,34.29 | v90.17,30.48 89.56,29.87 86.92,29.87 85.72,31.06 JP2.31
  Bottom 0.254: v77.75,51.46 78.74,50.47 v78.74,48.26 | v90.17,34.29 v90.17,30.48
GPIO13
  Top 0.254: U2.23 81.92,32.38 JP2.33
GPIO14
  Top 0.254: U2.22 80.64,31.11 JP2.35
GPIO15
  Top 0.254: U2.21 79.38,29.84 JP2.37
GPIO16  (via drill 0.35)
  Top 0.254: U2.8 v70.64,29.84
  Bottom 0.254: v70.64,29.84 77.5,29.84 85.11,22.23 87,22.23 JP2.38
GPIO17  (via drill 0.35)
  Top 0.254: U2.7 v70.64,31.11
  Bottom 0.254: v70.64,31.11 78.69,31.11 85.11,24.69 86.92,24.69 JP2.36
GPIO18  (via drill 0.35)
  Top 0.254: U2.6 v70.64,32.38
  Bottom 0.254: v70.64,32.38 79.98,32.38 85.09,27.28 86.97,27.28 JP2.34
GPIO19  (via drill 0.35)
  Top 0.254: U2.5 v70.66,33.66
  Bottom 0.254: v70.66,33.66 81.15,33.66 85.04,29.77 86.92,29.77 JP2.32
GPIO20  (via drill 0.35)
  Top 0.254: U2.4 v70.74,34.92
  Bottom 0.254: v70.74,34.92 82.53,34.92 85.06,32.38 87,32.38 JP2.30
GPIO21  (via drill 0.35)
  Top 0.254: U2.3 70.79,36.2 v70.81,36.22
  Bottom 0.254: v70.81,36.22 83.16,36.22 84.48,34.9 87,34.9 88.27,36.17 JP2.28
GPIO22  (via drill 0.35)
  Top 0.254: U2.2 v70.89,37.47
  Bottom 0.254: v70.89,37.47 87,37.47 JP2.26
GPIO23  (via drill 0.35)
  Top 0.254: U2.1 70.84,38.73 v70.87,38.71
  Bottom 0.254: v70.87,38.71 78.74,38.71 83.74,38.71 85.06,40.03 87.02,40.03 JP2.24
HV
  Top 1.016: JP1.17 JP1.18
I2C_SCL  (via drill 0.35)
  Top 0.203: JP1.1 7.7,68.5 U3.4
  Top 0.305: v45.72,38.1 44.68,38.1 R3.1 v44.45,40.64 | v55.02,40.44 54.86,40.59 U1.40
  Bottom 0.305: v45.72,38.1 53.34,38.1 55.02,39.78 v55.02,40.44 | JP1.1 6.99,67.94 6.35,67.31 6.35,59.69 7.01,59.03 12.09,59.03 12.7,58.42 12.7,57.15 13.97,55.88 33.02,55.88 34.29,54.61 34.29,45.72 38.1,41.91 43.18,41.91 v44.45,40.64
I2C_SDA  (via drill 0.35)
  Top 0.203: v5.08,59.69 5.08,69.85 v6.35,71.12 | v11.43,71.12 12.62,72.31 U3.5
  Top 0.305: R4.1 v41.91,40.01 | v54.36,40.01 U1.39 | v5.08,59.69 5.71,60.33 JP1.7
  Bottom 0.203: v6.35,71.12 v11.43,71.12
  Bottom 0.305: v54.36,40.01 v41.91,40.01 41.27,40.64 38.1,40.64 33.02,45.72 33.02,53.34 31.75,54.61 12.72,54.61 12.14,54.03 6.93,54.03 5.08,55.88 v5.08,59.69
IO_EXP_CS  (via drill 0.35)
  Top 0.254: U1.51 61.95,44.73 v62.23,44.45 | v65.28,30.53 67.26,30.53 v67.31,30.48 | v67.31,26.67 67.94,26.04 U2.11
  Bottom 0.254: v62.23,44.45 62.79,43.89 62.79,32.16 64.41,30.53 v65.28,30.53 | v67.31,30.48 v67.31,26.67
IO_EXP_INT_A  (via drill 0.35)
  Top 0.254: U1.53 62.17,45.73 v62.23,45.78 | v67.31,43.18 v71.12,43.18 | U2.20 73.03,28.57 72.39,29.21 v72.39,39.37
  Bottom 0.254: v62.23,45.78 62.29,45.72 66.04,45.72 67.31,44.45 v67.31,43.18 | v71.12,43.18 72.39,41.91 v72.39,39.37
MCU_RESET  (via drill 0.35)
  Top 0.203: U1.52 62.42,45.23 63.82,43.83 C13.2
  Top 0.254: v72.39,15.24 74.27,15.24 R7.1 | C13.2 63.82,41.59 v66.04,39.37 | R12.1 v66.04,16.99 | v66.04,16.99
  Bottom 0.254: v66.04,39.37 v66.04,16.99 66.04,16.51 67.31,15.24 v72.39,15.24
MOSI  (via drill 0.35)
  Top 0.203: v59.47,44.32 v59.47,41.94 | v65.13,23.52 69.11,23.52 U2.13 | v60.02,25.3 61.32,24 v62.33,24
  Top 0.254: U1.25 51.04,47.23 v51.33,47.52
  Top 0.305: R1.1 46.35,46.35 47.23,47.23 U1.25
  Bottom 0.203: v59.47,41.94 59.47,25.85 v60.02,25.3 | v65.13,23.52 62.81,23.52 v62.33,24
  Bottom 0.254: v59.47,44.32 59.34,44.45 55.5,44.45 52.51,47.43 52.43,47.52 v51.33,47.52
N$1  (via drill 0.35)
  Top 0.305: R5.1 44.22,76.2 v41.91,76.2 | v38.51,76.83 MICRO_SD.7
  Bottom 0.305: v41.91,76.2 39.14,76.2 v38.51,76.83
N$2
  Top 0.406: C15.1 49.51,18.68 R8.2 | R8.2 52.02,18.64 U4.1 | R8.2 49.55,13.62 U$7.SH1 49.56,12.21 U$7.SH3 U$7.SH4 U$7.SH5 U$7.SH6 56.47,11.05 U$7.SH2
N$3
  Top 0.508: JP1.16 18.4,50.16 F3.1
  Top 1.016: JP1.15 JP1.16
N$4
  Top 0.254: R10.1 DEBUG1.A
N$5
  Top 0.203: R11.1 81.28,11.43 80.51,10.66 STATUS.P6
N$6
  Top 0.508: USB_POWER.1 29.8,45.06 U5.4 U5.2 C17.1
N$7
  Top 0.254: R9.1 DEBUG0.A
N$8
  Top 0.203: R13.1 85.09,11.43 83.82,10.16 82.55,10.16 81.28,8.89 STATUS.P5
N$9
  Top 0.203: R14.1 88.9,10.16 86.36,7.62 82.55,7.62 82.05,7.12 STATUS.P4
RESET
  Top 0.305: R7.2 73.76,10.16 64.77,10.16 63.5,11.43 SWD.P10
RX0  (via drill 0.35)
  Top 0.254: U1.14 52.36,50.79 v52.38,50.77 | v14.99,39.88 10.92,39.88 JP1.24 | v39.93,49.51 36.88,49.51 v32.44,45.06
  Bottom 0.254: v52.38,50.77 51.13,49.53 39.95,49.53 v39.93,49.51 | v14.99,39.88 30.53,39.88 31.52,40.87 31.75,41.1 32.44,41.78 v32.44,45.06
RX1  (via drill 0.35)
  Top 0.254: U1.36 52.86,36.58 v51.84,35.56
  Bottom 0.254: v51.84,35.56 12.7,35.56 12.06,34.92 JP1.28
RX2  (via drill 0.35)
  Top 0.254: U1.30 48.54,44.73 48.26,44.45 48.26,43.18 46.99,41.91 42.04,41.91 v34.92,34.8
  Bottom 0.254: v34.92,34.8 29.97,29.84 JP1.32
RX3
  Top 0.254: U1.44 56.86,30.19 51.44,24.77 31.75,24.77 | 31.75,24.77 JP1.36 | SERIAL.2 31.75,24.77
SCK  (via drill 0.35)
  Top 0.203: v65.15,24.77 U2.12
  Top 0.254: U1.26 51.27,46.73 v51.36,46.63
  Top 0.305: R2.1 46.35,43.81 46.99,44.45 46.99,45.72 48,46.73 U1.26
  Bottom 0.203: v65.15,24.77 64.14,24.77 62.23,26.67 62.23,41.86 60.38,43.71 55.6,43.71 52.68,46.63 v51.36,46.63
SD_CS
  Top 0.254: U1.20 47.55,49.73 46.99,50.29 46.99,78.74 45.72,80.01 34.29,80.01 33.01,78.73 MICRO_SD.2
SD_DETECT  (via drill 0.35)
  Top 0.254: U2.25 82.73,34.92 85.22,32.44 92.13,32.44 v92.71,33.02 | v34.9,64.19 34.38,64.7 MICRO_SD.10
  Bottom 0.254: v92.71,33.02 92.71,69.85 91.44,71.12 49.53,71.12 41.91,63.5 35.56,63.5 34.9,64.16 v34.9,64.19
SPI_MISO  (via drill 0.35)
  Top 0.203: v65.13,22.28 69.09,22.28 U2.14
  Top 0.254: U1.27 50.86,46.23 v51.44,45.65
  Top 0.305: U1.27 48.36,46.23 v47.65,45.52 | v35.56,59.69 36.83,60.96 40.64,60.96 44.45,64.77 R5.2
  Bottom 0.203: v65.13,22.28 62.81,22.28 60.96,24.13 60.96,41.91 59.69,43.18 55.58,43.18 53.19,45.57 53.11,45.65 v51.44,45.65
  Bottom 0.305: v47.65,45.52 45.31,43.18 39.37,43.18 36.83,45.72 36.83,55.88 34.29,58.42 | 34.29,58.42 15.24,58.42 13.31,60.35 10.82,60.35 JP1.8 | 34.29,58.42 v35.56,59.69
SPI_MOSI  (via drill 0.35)
  Top 0.305: R1.2 40.01,46.35 v39.37,46.99 | v34.09,76.83 34.09,77.99 MICRO_SD.3
  Bottom 0.305: v39.37,46.99 39.06,47.3 39.06,61.27 37.47,62.87 34.29,62.87 | 34.29,62.87 JP1.6 | 34.29,62.87 34.09,63.07 v34.09,76.83
SPI_SCK  (via drill 0.35)
  Top 0.305: R2.2 40.01,43.81 v39.37,44.45 | v15.24,60.96 13.97,62.23 13.97,67.31 13.34,67.94 JP1.2 | MICRO_SD.5 36.31,76.8 v36.3,76.78 | v36.3,61.85 v36.3,65.1
  Bottom 0.305: v39.37,44.45 37.92,45.9 37.92,59.87 36.83,60.96 36.27,60.96 | 36.27,60.96 v15.24,60.96 | v36.3,61.85 36.3,60.98 36.27,60.96 | v36.3,65.1 v36.3,76.78
STAT_B  (via drill 0.35)
  Top 0.254: U2.24 76.83,33.66 76.2,33.02 v76.2,29.21 | v76.2,27.94 76.2,26.67 75.82,26.29 75.82,24.59 76.2,24.21 76.2,21.59 81.28,16.51 R11.2
  Bottom 0.254: v76.2,29.21 v76.2,27.94
STAT_G  (via drill 0.35)
  Top 0.254: U2.26 76.83,36.2 74.93,34.29 v74.93,29.21 | v74.93,27.94 74.93,21.59 v76.2,20.32 | v80.01,20.32 82.55,20.32 85.09,17.78 R13.2
  Bottom 0.254: v74.93,29.21 v74.93,27.94 | v76.2,20.32 v80.01,20.32
STAT_R  (via drill 0.35)
  Top 0.254: U2.27 74.3,37.47 73.66,36.83 v73.66,29.21 | v73.66,27.94 73.66,20.32 74.93,19.05 v76.2,19.05 | v86.36,19.05 88.9,16.51 R14.2
  Bottom 0.254: v73.66,29.21 v73.66,27.94 | v76.2,19.05 v86.36,19.05
SWDCLK  (via drill 0.35)
  Top 0.254: R6.1 71.6,18.57 v69.85,20.32 | v58.42,48.06 58.75,47.73 U1.57
  Top 0.305: R6.1 71.6,11.91 70.59,10.9 68.1,10.9 67.31,11.68 SWD.P4
  Bottom 0.254: v69.85,20.32 69.85,46.28 68.45,47.68 58.8,47.68 v58.42,48.06
SWDIO  (via drill 0.35)
  Top 0.254: v69.55,16.05 69.55,12.39 69.22,12.06 SWD.P2 | v68.68,48.26 68.66,48.23 v68.66,45.72 | v59.08,48.56 59.42,48.23 U1.58
  Bottom 0.254: v69.55,16.05 68.66,16.94 v68.66,45.72 | v68.68,48.26 68.38,48.56 v59.08,48.56
TX0  (via drill 0.35)
  Top 0.254: U1.13 52.86,51.76 v53.09,51.54 | v39.85,51.51 38.33,49.99 35.61,49.99 31.65,46.02 v31.65,44.22 | JP1.26 14.61,37.47 v17.78,40.64
  Bottom 0.254: v53.09,51.54 39.88,51.54 v39.85,51.51 | v31.65,44.22 31.65,41.81 30.48,40.64 v17.78,40.64
TX1
  Top 0.254: U1.35 52.36,37.12 47.62,32.38 JP1.30
TX2  (via drill 0.35)
  Top 0.254: U1.29 48.5,45.23 47.88,44.61 47.88,44.07 46.23,42.42 39.09,42.42 v31.52,34.85 | v27.58,30.89 24,27.3 JP1.34
  Bottom 0.254: v31.52,34.85 27.58,30.91 v27.58,30.89
TX3  (via drill 0.35)
  Top 0.254: U1.43 56.36,30.96 50.8,25.4 v29.21,25.4 v13.97,25.4
  Bottom 0.254: v13.97,25.4 12.7,24.13 12.7,22.86 12.06,22.23 JP1.38 | SERIAL.3 v29.21,25.4
USB_D+
  Top 0.254: U1.46 57.86,26.11 53.34,21.59 53.34,16.97 | 53.34,16.97 53.34,13.06 U$7.3 | U4.3 53.35,16.96 53.34,16.97
USB_D-
  Top 0.254: U1.45 57.36,26.15 52.72,21.5 52.72,16.99 | U$7.2 52.72,16.99 | U4.2 52.68,16.96 52.72,16.99
V_BATT
  Top 1.016: JP1.9 JP1.10 | JP1.10 JP1.12 | JP1.12 JP1.11 | JP1.11 JP1.9 | JP1.9 JP1.12 | JP1.11 JP1.10
V_USB  (via drill 0.35)
  Top 0.406: U$7.1 v52.07,15.24 | v54.61,20.32 55.04,19.89 55.04,19.36 54.54,18.86 U4.4 | v48.26,22.86 46.99,22.86 45.72,24.13 v40.64,24.13 | v34.29,33.02 v27.94,33.02 | v26.67,34.29 26.67,38.69 C16.1 24.12,38.73 24.11,38.72
  Top 0.508: 24.11,38.72 U5.3
  Bottom 0.406: 52.07,20.32 v52.07,15.24 36.83,15.24 SERIAL.1 | 52.07,20.32 v54.61,20.32 | 52.07,20.32 52.07,21.59 50.8,22.86 v48.26,22.86 | v40.64,24.13 38.1,26.67 38.1,30.48 35.56,33.02 v34.29,33.02 | v27.94,33.02 v26.67,34.29
VCC_MCU_3V3  (via drill 0.35)
  Top 0.254: C2.1 47.94,39.05 45.72,36.83 45.72,35.97 45.26,35.51 44.63,35.51 R3.2 R4.2 | C13.1 67.31,44.77 v67.31,45.72 | v63.91,46.94 63.66,47.19 63.66,48.1
  Top 0.305: C2.1 50.48,39.05 51.86,40.43 U1.34 51.86,43.12 52.4,43.66 52.4,49.23 | C1.1 U1.21 52.4,49.23 | 52.4,49.23 56.18,49.23 58.18,47.23 | 58.18,47.23 U1.56 62.79,47.23 63.66,48.1 C4.1 | 58.18,47.23 58.86,46.55 U1.48 C3.1 | C3.1 | C3.1 58.86,37.66 59.69,36.83 63.5,36.83 64.32,36.01 C12.1 64.32,19.85 R12.2 65.25,19.84 67.36,17.73 R6.2 68.61,13.36 SWD.P1
  Top 0.406: C12.1 U2.9 70.56,28.57 v70.59,28.55 | MICRO_SD.4 v35.2,79.35 | v26.67,79.35 26.01,79.35 25.38,78.72 C11.1 22.86,77.61 | 22.86,77.61 C14.+ 8.46,77.6 U3.1 | 22.86,77.61 22.86,54.61 24.33,53.14 L1.2 | v76.71,26.04 U2.18
  Top 0.508: FB1.1 40.83,53.22 40.83,53.17 | 40.83,53.17 40.83,50.43 42.01,49.25 C1.1 | L1.2 C8.1 40.8,53.14 40.83,53.17
  Bottom 0.254: v67.31,45.72 66.09,46.94 v63.91,46.94
  Bottom 0.406: v35.2,79.35 v26.67,79.35 | v70.59,28.55 73.1,26.04 v76.71,26.04
VCC_MCU_ANA  (via drill 0.35)
  Top 0.305: C7.1 55.35,53.16 U1.8
  Top 0.508: FB1.2 41.92,55.88 C6.1 v46.35,55.88
  Bottom 0.508: C7.1 arc45 55.26,55.88 v46.35,55.88
  other vias: 55.35,55.84
VCC_MCU_CORE
  Top 0.254: U1.55 62.81,46.73 C5.1
XIN32
  Top 0.305: C9.2 63.69,55.37 XTAL1.P$1 60.2,55.19 58.86,53.86 U1.1
XOUT32
  Top 0.305: U1.2 58.36,54.55 XTAL1.P$2 59.18,56.59 60.35,57.76 60.38,57.78 C10.2

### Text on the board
tPlace: BOARD # / 1 2 3 4 | REV B | MCU
tNames: CU InSpace | MCU Board - 2019 | Samuel Dewan | GND | TXD | RXD | VUSB | DEBUG 0 | DEBUG 1

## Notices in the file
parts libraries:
SparkFun-PowerSymbols: Licensing: Creative Commons ShareAlike 4.0 International - https://creativecommons.org/licenses/by-sa/4.0
